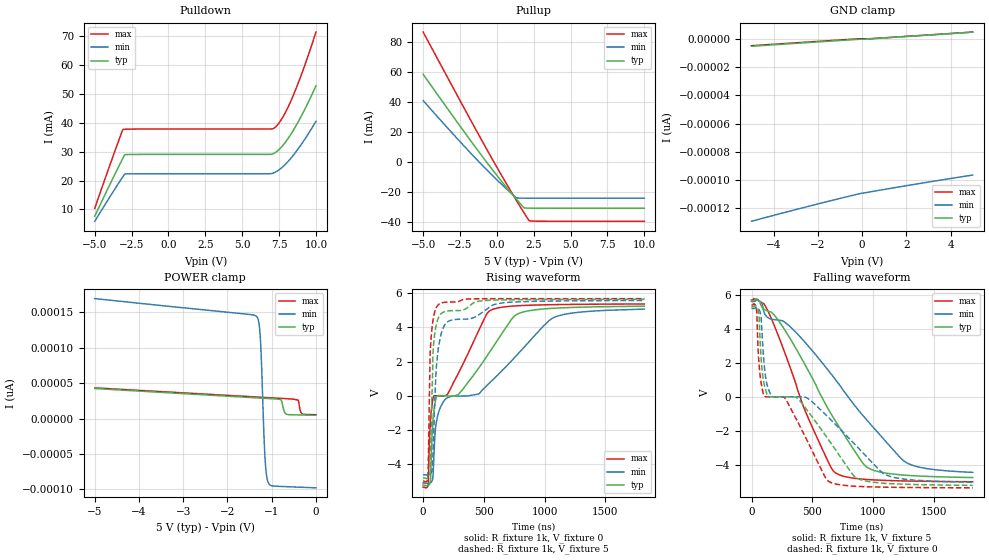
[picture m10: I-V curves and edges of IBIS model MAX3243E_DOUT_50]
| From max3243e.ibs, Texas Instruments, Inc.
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[Model]   MAX3243E_DOUT_50
Model_type  3-state
Enable   Active-High
Vref =   0
Rref =   3000
Cref =   150p
Vmeas =   1.5
| variable   typ   min   max
C_comp   3.66pF   3.03pF   4.14pF
| C_pullup   3.99pF   3.02pF   4.95pF
| C_pulldown   3.82pF   2.73pF   5.25pF
| C_tri-state   3.66pF   3.03pF   4.14pF
[Temperature Range]   40   100   -40
| Ambient temperature   25   85   -40
[Voltage range]   5   4.5   5.5
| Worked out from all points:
|   slope of the pullup table from 0 to 0.75 V, typ, clamps not added: 81.7 ohm
|   rising waveform, R_fixture 1k, V_fixture 0: 20-80 % time 533ns typ, 764ns min, 370ns max; typ from -5.23 V to 5.24 V
|   falling waveform, R_fixture 1k, V_fixture 5: 20-80 % time 497ns typ, 689ns min, 346ns max; typ from 5.65 V to -4.73 V
|   rising waveform, R_fixture 1k, V_fixture 5: 20-80 % time 30.2ns typ, 60.3ns min, 22.3ns max; typ from -4.8 V to 5.64 V
|   falling waveform, R_fixture 1k, V_fixture 0: 20-80 % time 619ns typ, 784ns min, 449ns max; typ from 5.29 V to -5.19 V
[GND Clamp]
| MAX3243E_DOUT_50
|   Voltage   I(typ)   I(min)   I(max)
-5V       -5.152pA   -129.2pA   -4.796pA
-2.23V    -2.321pA   -117.9pA   -1.945pA
-295mV    -363.6fA   -110.3pA   8.016fA
-80mV     -202.2fA   -109.6pA   88.26fA
335mV     80.85fA    -108.5pA   163.4fA
2.52V     2.301pA    -102.7pA   2.368pA
5V        4.856pA    -96.45pA   4.912pA
[POWER Clamp]
| MAX3243E_DOUT_50
|   Voltage   I(typ)   I(min)   I(max)
-5V       42.54pA    169.5pA    43.47pA
-1.35V    29.38pA    144.9pA    30.62pA
-1.295V   29.18pA    137pA      30.42pA
-1.26V    29.05pA    116.4pA    30.3pA
-1.235V   28.96pA    85.08pA    30.21pA
-1.155V   28.68pA    -51.35pA   29.93pA
-1.085V   28.42pA    -89.26pA   29.68pA
-795mV    26.75pA    -95.7pA    28.66pA
-660mV    6.17pA     -96.05pA   28.19pA
-405mV    5.299pA    -96.69pA   26.08pA
-310mV    5.192pA    -96.92pA   6.7pA
-84.45fV  4.856pA    -97.69pA   5.537pA
[Pulldown]
| MAX3243E_DOUT_50
|   Voltage   I(typ)   I(min)   I(max)
-5V       7.69mA     5.923mA    10.43mA
-3.855V   19.91mA    15.32mA    27.06mA
-3.09V    27.77mA    21.36mA    37.69mA
-2.96V    28.93mA    22.24mA    37.76mA
-2.855V   29.01mA    22.33mA    37.77mA
6.85V     29.07mA    22.38mA    37.85mA
7.215V    29.6mA     22.84mA    38.37mA
7.465V    30.59mA    23.61mA    39.72mA
7.745V    32.1mA     24.76mA    41.87mA
8.385V    36.72mA    28.27mA    48.53mA
9.13V     43.52mA    33.45mA    58.29mA
10V       52.78mA    40.52mA    71.4mA
[Pullup]
| MAX3243E_DOUT_50
|   Voltage   I(typ)   I(min)   I(max)
-5V       58.59mA    41.03mA    86.78mA
-1.63V    12.26mA    4.437mA    25.34mA
-395mV    -3.918mA   -8.055mA   3.396mA
735mV     -17.91mA   -18.72mA   -15.93mA
1.355V    -25.17mA   -23.95mA   -26.12mA
1.855V    -30.57mA   -24.11mA   -34.08mA
2.195V    -30.8mA    -24.13mA   -39.16mA
10V       -30.87mA   -24.15mA   -39.56mA
[Ramp]
| MAX3243E_DOUT_50
| variable   typ   min   max
dV/dt_r   6.30/5.33E-07   6.12/7.63E-07   6.45/3.70E-07
dV/dt_f   6.27/5.00E-07   6.05/6.95E-07   6.45/3.48E-07
R_load = 1k
[Rising Waveform]
| MAX3243E_DOUT_50
R_fixture =   1k
C_fixture =   0
L_fixture =   0
V_fixture =   0
V_fixture_min = 0
V_fixture_max = 0
|   Time   V(typ)   V(min)   V(max)
0s        -5.226V    -5.098V    -5.343V
41.4ns    -5.242V    -5.129V    -5.173V
58.8ns    -5.012V    -5.096V    -1.636V
84.4ns    -1.159V    -4.257V    -70.98mV
105.7ns   -141.1mV   -1.686V    10.47mV
165ns     -3mV       -370.3mV   -7.5mV
541.6ns   2.499V     722mV      4.94V
760.4ns   4.718V     2.299V     5.262V
1.075us   5.124V     4.584V     5.334V
1.82us    5.244V     5.073V     5.375V
[Falling Waveform]
| MAX3243E_DOUT_50
R_fixture =   1k
C_fixture =   0
L_fixture =   0
V_fixture =   5
V_fixture_min = 4.5
V_fixture_max = 5.5
|   Time   V(typ)   V(min)   V(max)
0s        5.65V      5.593V     5.689V
58.3ns    5.663V     5.636V     5.658V
78.8ns    5.358V     5.555V     5.551V
136.8ns   5.029V     4.642V     5.013V
317.4ns   3.426V     4.122V     1.738V
452.8ns   1.727V     3.104V     -1.01V
684.7ns   -1.344V    1.074V     -4.416V
942.6ns   -4.079V    -1.307V    -4.839V
1.263us   -4.591V    -3.8V      -4.929V
1.82us    -4.731V    -4.427V    -4.976V
[Rising Waveform]
| MAX3243E_DOUT_50
R_fixture =   1k
C_fixture =   0
L_fixture =   0
V_fixture =   5
V_fixture_min = 4.5
V_fixture_max = 5.5
|   Time   V(typ)   V(min)   V(max)
0s        -4.805V    -4.616V    -4.995V
40.5ns    -4.801V    -4.639V    -4.659V
57.5ns    -4.401V    -4.582V    2.392V
75.9ns    848.5mV    -4.221V    4.148V
88.6ns    3.215V     -1.777V    4.715V
107.5ns   4.131V     1.499V     5.148V
128.5ns   4.603V     2.91V      5.351V
201.1ns   4.963V     4.328V     5.482V
606.8ns   5.607V     5.383V     5.683V
1.82us    5.645V     5.577V     5.688V
[Falling Waveform]
| MAX3243E_DOUT_50
R_fixture =   1k
C_fixture =   0
L_fixture =   0
V_fixture =   0
V_fixture_min = 0
V_fixture_max = 0
|   Time   V(typ)   V(min)   V(max)
0s        5.287V     5.186V     5.388V
41.1ns    5.299V     5.24V      5.171V
58.3ns    4.997V     5.152V     2.291V
100.2ns   880.9mV    2.249V     113.2mV
165.2ns   1.871mV    54.06mV    7.05mV
278.8ns   8.993mV    7.171mV    -101.1mV
629.4ns   -2.467V    -1.175V    -4.921V
852.9ns   -4.697V    -2.803V    -5.239V
1.108us   -5.072V    -4.579V    -5.296V
1.82us    -5.189V    -5.011V    -5.333V
